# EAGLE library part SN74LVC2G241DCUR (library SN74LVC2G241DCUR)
Dual Buffer/Driver With 3-State Outputs Source: Datasheet
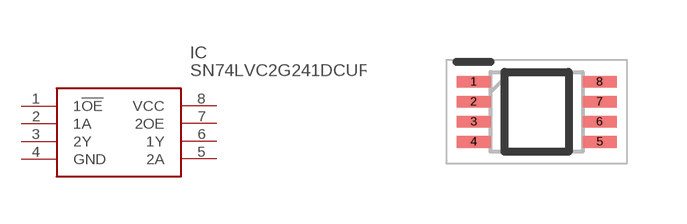
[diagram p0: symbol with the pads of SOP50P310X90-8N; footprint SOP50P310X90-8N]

Designator prefix IC

## SN74LVC2G241DCUR (Description: Dual Buffer/Driver With 3-State Outputs; Height: 0.9mm; Manufacturer_Name: Texas Instruments; Manufacturer_Part_Number: SN74LVC2G241DCUR; Mouser_Part_Number: 595-SN74LVC2G241DCUR; Mouser_Price-Stock: https://www.mouser.co.uk/ProductDetail/Texas-Instruments/SN74LVC2G241DCUR?qs=JS6RUWRH9DV7W1UO8b3P2w%3D%3D)  [SOP50P310X90-8N]
1  1!OE
2  1A
3  2Y
4  GND
5  2A
6  1Y
7  2OE
8  VCC

## Footprint SOP50P310X90-8N (pad centres in mm)
DCU (R-PDSO-G8)
smd 0.85 x 0.3: 1 -1.575,0.75; 2 -1.575,0.25; 3 -1.575,-0.25; 4 -1.575,-0.75; 5 1.575,-0.75; 6 1.575,-0.25; 7 1.575,0.25; 8 1.575,0.75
